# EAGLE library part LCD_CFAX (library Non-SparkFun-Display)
Graphic LCD module (LCD-00463) DISCONTINUED
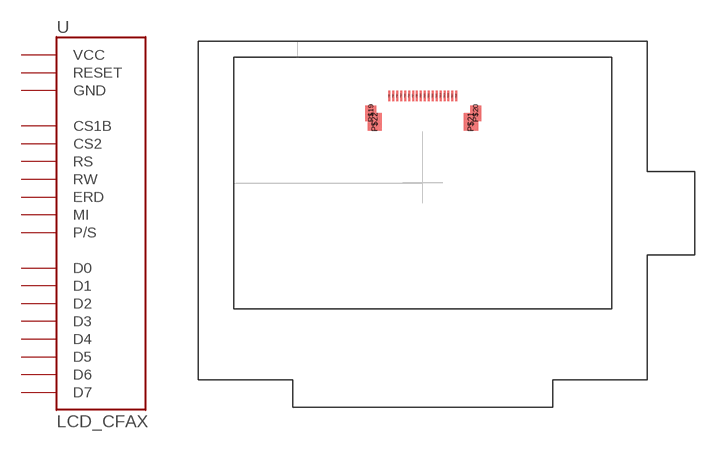
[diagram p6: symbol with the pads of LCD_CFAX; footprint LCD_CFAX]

Designator prefix -

## LCD_CFAX  [LCD_CFAX]
P$1  VCC
P$2  GND
P$3  CS1B
P$4  CS2
P$5  RESET
P$6  RS
P$7  RW
P$8  ERD
P$9  D0
P$10  D1
P$11  D2
P$12  D3
P$13  D4
P$14  D5
P$15  D6
P$16  D7
P$17  MI
P$18  P/S

## Footprint LCD_CFAX (pad centres in mm)
CFAX LCD (crystalfontz) For 128x64 LCDs. Specifications: Pin count: 16 Pin pitch: 0.1" Area: Datasheet referenced for footprint: Example device(s): CrystalFontz LCD
smd 0.25 x 1.3: P$1 -4.25,11.05; P$2 -3.75,11.05; P$3 -3.25,11.05; P$4 -2.75,11.05; P$5 -2.25,11.05; P$6 -1.75,11.05; P$7 -1.25,11.05; P$8 -0.75,11.05; P$9 -0.25,11.05; P$10 0.25,11.05; P$11 0.75,11.05; P$12 1.25,11.05; P$13 1.75,11.05; P$14 2.25,11.05; P$15 2.75,11.05; P$16 3.25,11.05; P$17 3.75,11.05; P$18 4.25,11.05
smd 1.4 x 2: P$19 -6.6,8.85; P$20 6.7,8.85
smd 1.8 x 2.2: P$21 6.1,7.75; P$22 -6.1,7.75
